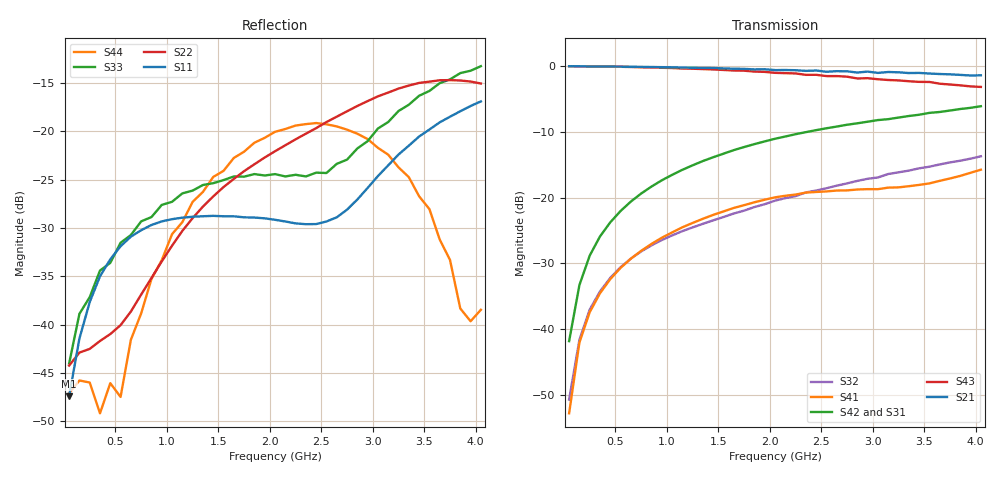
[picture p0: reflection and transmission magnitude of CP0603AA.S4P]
! Network Analyzer HP8720D.07.14 Serial No. US38111185
! 28 Apr 1999  02:06:29
! Frequency 	S11		S21		S31		S41		S12		S22		S23		S24		S13		S23		S33		S34		S14		S24		S34		S44
# HZ  S  DB R 50
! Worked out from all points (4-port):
!   41 points, 50 MHz to 4.05 GHz, reference 50 ohm
!   strongest paths, dB at 50 MHz, 1.05 GHz, 2.05 GHz, 3.05 GHz, 4.05 GHz:
!     S21: 0.0, -0.2, -0.6, -1.0, -1.4
!     S43: 0.0, -0.3, -1.0, -2.0, -3.2
!     S42: -41.8, -16.5, -11.0, -8.2, -6.1
!     S31: -42.1, -16.5, -11.1, -8.3, -6.2
!     S41: -52.8, -25.3, -19.9, -18.7, -15.7
!     S32: -50.7, -25.7, -20.5, -16.9, -13.7
!   lowest |S11| = -47.4 dB at 50 MHz (marker M1), VSWR 1.01, Z = 50.4 - j0.228 ohm
!   |S11| at or under -10 dB: start of sweep to end of sweep
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5e7  -47.43 -32.1  -0.02 -1.1  -42.34 86.2  -49.90 95.0
     -0.01 -1.0  -44.24 18.1  -51.24 77.9  -43.88 94.3
     -42.13 92.0  -50.70 96.7  -44.03 17.3  -0.02 -1.3
     -52.79 91.8  -41.82 88.5  -0.00 -1.1  -47.10 -1.4
2.5e8  -37.67 -78.9  -0.03 -4.7  -28.75 84.2  -37.42 85.4
       -0.04 -4.9  -42.52 7.9  -37.17 83.8  -28.80 84.5
       -28.77 84.1  -37.03 83.8  -37.16 51.0  -0.03 -5.7
       -37.41 84.5  -28.81 84.3  -0.03 -5.8  -46.00 -31.1
5.5e8  -31.88 -103.9  -0.08 -10.3  -21.96 78.0  -30.70 78.5
       -0.07 -10.5  -40.06 17.8  -30.60 75.6  -22.03 78.3
       -21.98 77.8  -30.57 75.7  -31.52 63.1  -0.10 -12.5
       -30.67 78.4  -22.02 78.2  -0.10 -12.6  -47.49 -119.5
1.25e9  -28.83 -142.6  -0.22 -23.3  -15.05 63.5  -23.80 65.6
        -0.23 -23.7  -28.97 24.0  -24.50 63.7  -15.09 64.1
        -15.09 63.3  -24.52 63.9  -26.12 71.8  -0.40 -27.8
        -23.84 65.4  -15.08 64.1  -0.39 -28.2  -27.29 169.8
2.25e9  -29.52 157.2  -0.58 -41.7  -10.36 42.6  -19.38 44.1
        -0.61 -42.5  -20.82 -10.6  -19.65 51.7  -10.53 44.8
        -10.53 43.0  -19.75 52.8  -24.49 46.0  -1.08 -48.9
        -19.52 44.6  -10.34 43.6  -1.11 -49.6  -19.39 143.8
3.15e9  -23.51 51.6  -0.89 -59.0  -8.02 24.6  -18.43 32.4
        -0.89 -57.2  -15.97 -31.4  -16.37 37.2  -8.27 28.2
        -7.99 26.6  -16.40 39.4  -19.02 -39.6  -1.88 -66.5
        -18.47 34.0  -8.06 26.5  -2.10 -66.3  -22.41 111.0
4.05e9  -16.89 20.8  -2.20 -76.3  -6.51 4.4  -15.77 27.3
        -1.39 -73.5  -15.04 -55.5  -13.76 15.1  -6.45 13.3
        -6.20 11.5  -13.70 21.7  -13.24 -88.8  -3.07 -88.7
        -15.74 33.0  -6.09 12.3  -3.16 -82.1  -38.47 -58.1
